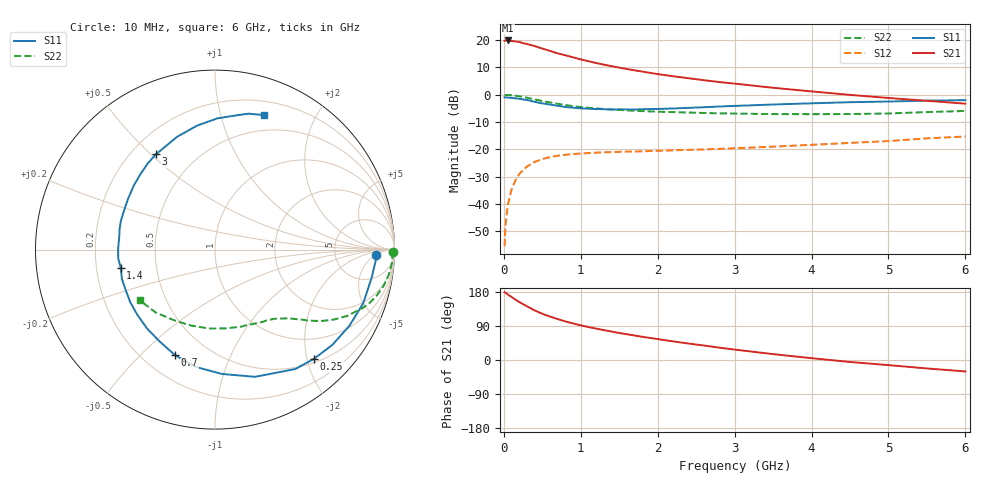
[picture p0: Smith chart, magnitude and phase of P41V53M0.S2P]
! SIEMENS Small Signal Semiconductors
! BFP182
! Si NPN RF Bipolar Junction Transistor in SOT143
! VCE = 1.5 V  IC = 3 mA
! Common Emitter S-Parameters:  March  1996
# GHz  S  MA  R  50
!  f  S11  S21  S12  S22
! GHz  MAG  ANG  MAG  ANG  MAG  ANG  MAG  ANG
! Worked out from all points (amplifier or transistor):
!   36 points, 10 MHz to 6 GHz, reference 50 ohm
!   highest |S21| = 19.9 dB at 50 MHz (marker M1)
!   |S21| within 3 dB of that: start of sweep to 503.5 MHz
!   unconditionally stable (mu >= 1): 1.874 GHz to 5.955 GHz
!   at 250 MHz: K = 0.16, MSG = 23.2 dB, |S12| = -27.6 dB
!   at 1.4 GHz: K = 0.80, MSG = 15.7 dB, |S12| = -21.0 dB
!   at 6 GHz: K = 1.00, MSG = 6.0 dB, |S12| = -15.3 dB
!   S11 on the Smith chart (normalised r, x): 10 MHz: 17, -5; 250 MHz: 0.57, -2.13; 700 MHz: 0.33, -0.64; 1.4 GHz: 0.31, -0.09; 3 GHz: 0.30, +0.52; 6 GHz: 0.33, +1.37
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0.01  0.8951 -1.9  9.723 179.0  0.0017 83.8  0.9937 -0.8
0.02  0.8975 -4.0  9.836 177.8  0.0039 85.5  0.9881 -1.6
0.05  0.8868 -10.0  9.846 173.1  0.0095 87.7  0.9894 -4.1
0.15  0.8609 -29.5  9.447 159.6  0.027 73.0  0.9614 -12.0
0.2  0.8424 -39.0  9.242 153.0  0.0354 68.2  0.9385 -15.6
0.25  0.8212 -47.8  8.783 147.2  0.0419 63.6  0.9119 -19.0
0.3  0.8018 -56.1  8.482 141.9  0.0485 59.5  0.8833 -21.7
0.4  0.7432 -72.5  7.779 130.9  0.059 52.2  0.8231 -26.7
0.5  0.6939 -86.8  6.994 122.0  0.0665 46.0  0.7678 -30.5
0.6  0.6625 -99.3  6.346 114.6  0.0727 41.1  0.7228 -33.3
0.7  0.6287 -110.8  5.721 108.0  0.0767 37.2  0.6824 -35.6
0.8  0.5973 -121.2  5.269 101.8  0.0799 33.8  0.6486 -37.5
0.9  0.5803 -130.6  4.838 96.5  0.0824 31.5  0.6186 -39.0
1.1  0.5558 -148.1  4.112 86.9  0.0858 27.6  0.5773 -41.8
1.4  0.5349 -169.0  3.331 75.1  0.0892 23.6  0.5387 -45.5
1.8  0.5433 168.1  2.655 61.2  0.0925 21.8  0.5024 -50.5
2.2  0.5608 149.9  2.184 49.1  0.0962 21.0  0.4823 -56.5
3  0.625 121.6  1.599 27.5  0.1051 20.7  0.4531 -71.3
3.5  0.6632 108.5  1.342 15.5  0.1123 20.5  0.443 -82.1
4.5  0.7308 89.1  0.995 -5.2  0.1316 19.1  0.4436 -107.3
5.5  0.7803 76.1  0.776 -22.3  0.1596 16.2  0.4818 -133.4
6  0.7969 70.1  0.687 -30.2  0.1722 12.6  0.5056 -146.1
